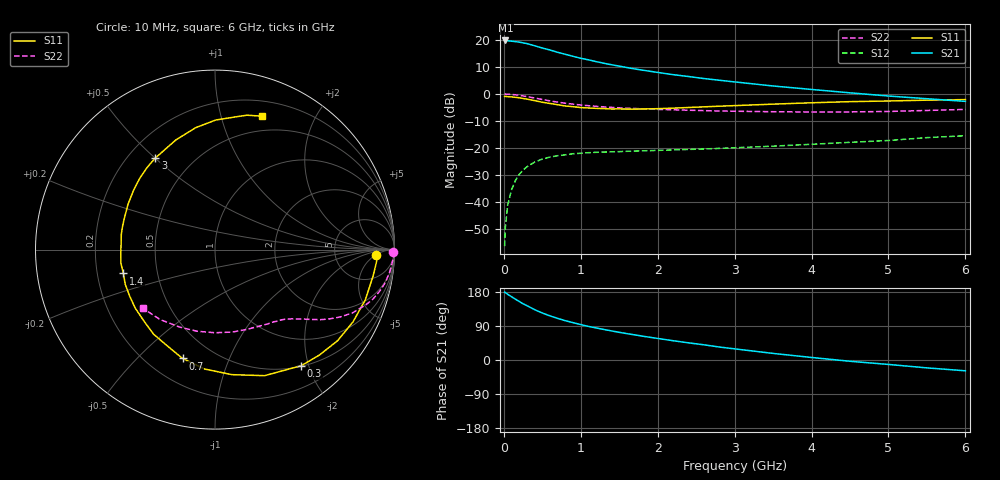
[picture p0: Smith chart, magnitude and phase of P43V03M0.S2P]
! SIEMENS Small Signal Semiconductors
! BFP182
! Si NPN RF Bipolar Junction Transistor in SOT143
! VCE = 3 V  IC = 3 mA
! Common Emitter S-Parameters:  March  1996
# GHz  S  MA  R  50
!  f  S11  S21  S12  S22
! GHz  MAG  ANG  MAG  ANG  MAG  ANG  MAG  ANG
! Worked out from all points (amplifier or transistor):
!   36 points, 10 MHz to 6 GHz, reference 50 ohm
!   highest |S21| = 19.9 dB at 20 MHz (marker M1)
!   |S21| within 3 dB of that: start of sweep to 526.1 MHz
!   unconditionally stable (mu >= 1): 1.925 GHz to 5.722 GHz
!   at 250 MHz: K = 0.15, MSG = 23.6 dB, |S12| = -28.2 dB
!   at 1.4 GHz: K = 0.78, MSG = 16.2 dB, |S12| = -21.5 dB
!   at 6 GHz: K = 0.97, MSG = 6.4 dB, |S12| = -15.5 dB
!   S11 on the Smith chart (normalised r, x): 10 MHz: 17, -5; 300 MHz: 0.51, -1.88; 700 MHz: 0.34, -0.69; 1.4 GHz: 0.31, -0.12; 3 GHz: 0.31, +0.50; 6 GHz: 0.34, +1.35
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0.01  0.8989 -1.8  9.735 178.9  0.0015 88.8  0.9942 -0.7
0.02  0.9039 -3.8  9.865 177.9  0.0034 81.5  0.9973 -1.5
0.05  0.8932 -9.4  9.74 173.4  0.0087 87.4  0.9914 -3.7
0.15  0.8679 -27.7  9.398 160.6  0.0247 74.2  0.9663 -11.0
0.2  0.8509 -36.6  9.191 154.4  0.0322 69.9  0.9461 -14.2
0.25  0.8271 -45.2  8.899 148.4  0.0387 65.6  0.9222 -17.4
0.3  0.8058 -53.4  8.63 143.4  0.0446 61.1  0.8951 -20.1
0.4  0.7549 -68.5  7.872 132.9  0.0545 54.3  0.8434 -24.7
0.5  0.7031 -82.3  7.138 124.0  0.0621 47.9  0.792 -28.3
0.6  0.6677 -95.1  6.566 116.4  0.0676 42.8  0.7453 -31.2
0.7  0.6327 -106.6  5.935 109.8  0.0716 39.0  0.7071 -33.5
0.8  0.5989 -116.3  5.457 103.7  0.0744 35.6  0.6739 -35.3
0.9  0.5825 -126.0  5.009 98.5  0.0779 33.1  0.6487 -36.8
1.1  0.5512 -143.8  4.307 88.6  0.0815 29.2  0.6072 -39.5
1.4  0.5276 -165.4  3.495 76.8  0.0846 25.3  0.5654 -43.2
1.8  0.5287 170.9  2.778 63.0  0.0883 23.2  0.532 -48.0
2.2  0.5469 152.3  2.288 50.9  0.0917 22.4  0.51 -53.8
3  0.609 123.1  1.677 29.4  0.1006 22.5  0.4794 -67.9
3.5  0.6489 109.6  1.409 17.4  0.1078 22.1  0.4692 -78.2
4.5  0.7219 89.7  1.052 -3.4  0.1269 21.1  0.4657 -102.4
5.5  0.7695 76.7  0.818 -20.8  0.1551 18.4  0.4955 -128.2
6  0.7878 70.7  0.73 -28.5  0.1681 14.8  0.5177 -140.8
